(* 	
	Program Name: 	ACS_DRIVE_OUTPUT_SCAN
	Purpose:		Copy Drive Outputs from shadow memory to output registers
*)
PROGRAM ACS_DRIVE_OUTPUT_SCAN
VAR_IN_OUT
	Axis:ACS_DRIVE_TYPE;
END_VAR

//Run Input Scan Sub Routines
ACS_WRITE_AXIS_BITS( Axis:= Axis);
ACS_WRITE_AXIS_VARIABLES(Axis:= Axis);

END_PROGRAM
